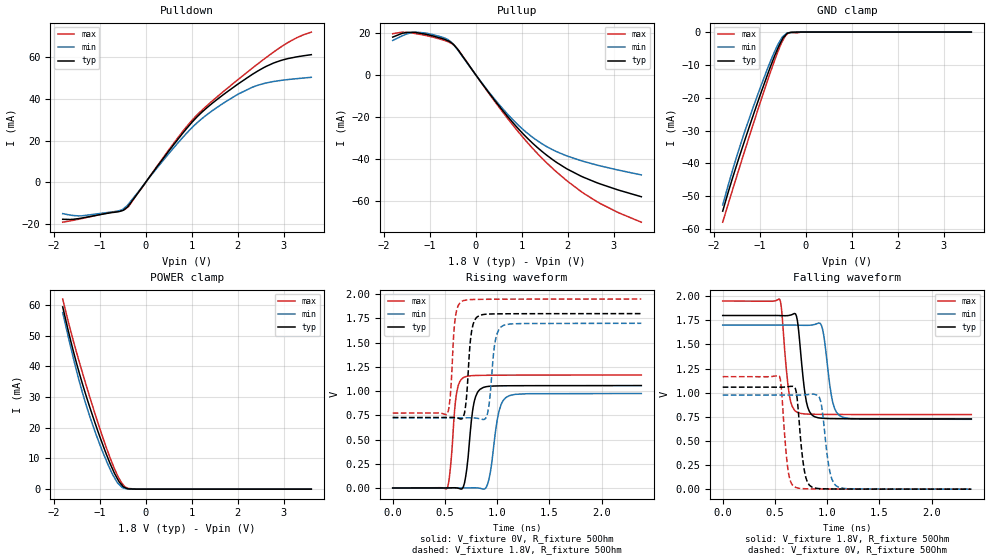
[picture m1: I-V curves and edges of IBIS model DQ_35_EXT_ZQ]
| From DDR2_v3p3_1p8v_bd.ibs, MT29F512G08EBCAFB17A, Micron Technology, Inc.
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| MODEL DQ_35_EXT_ZQ (35 Ohm Data I/O with no ODT, With ZQ Cal)
[Model]   DQ_35_EXT_ZQ
Model_type   I/O
Vinl = 650.000mV
Vinh = 1.150V
Vmeas = 900.000mV
Vref = 900.000mV
Cref = 0.0pF
Rref = 50.000Ohm
|   typ   min   max
|C_comp   1.200pF   1.100pF   1.300pF
C_comp_pullup   0.6000pF   0.5500pF   0.6500pF
C_comp_pulldown   0.6000pF   0.5500pF   0.6500pF
[Model Spec]
| Input threshold voltage corners
Vinl   0.6500V   0.6000V   0.7250V
Vinh   1.1500V   1.1000V   1.2250V
| Measurement voltage corners
Vmeas   0.9000V   0.8500V   0.9750V
| Timing spec test load voltage corners
Vref   0.9000V   0.8500V   0.9750V
| Dynamic Overshoot Parameters from ONFI4 Specification
D_overshoot_ampl_h   1.00   NA   NA
D_overshoot_ampl_l   1.00   NA   NA
D_overshoot_area_h   0.75n   NA   NA
D_overshoot_area_l   0.75n   NA   NA
[Receiver Thresholds]
Vth   =  0.900V
Vth_min  =  0.8820V
Vth_max  =  0.9180V
Vinh_ac  =  0.250V
Vinh_dc  =  0.125V
Vinl_ac  = -0.250V
Vinl_dc  = -0.125V
Tslew_ac =  5.000ns |Not specified, so set to high value
Threshold_sensitivity = 0.50
Reference_supply Pullup_ref
[Voltage Range]   1.8000V   1.7000V   1.9500V
[Pullup Reference]   1.8000V   1.7000V   1.9500V
| Junction Temperature (Ambient temp is 35C typ, 70C min, 0C max)
[Temperature Range]   50.0   85.0   0.0
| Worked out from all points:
|   slope of the pulldown table from 0 to 0.27 V, typ, clamps not added: 33.1 ohm
|   slope of the pullup table from 0 to 0.27 V, typ, clamps not added: 33.4 ohm
|   GND clamp passes 1 mA (typ) near -0.44 V on its own axis
|   POWER clamp passes 1 mA (typ) near -0.50 V on its own axis
|   falling waveform, V_fixture 1.8V, R_fixture 50Ohm: 20-80 % time 63.1ps typ, 71ps min, 58.7ps max; typ from 1.8 V to 0.728 V
|   rising waveform, V_fixture 0V, R_fixture 50Ohm: 20-80 % time 61.4ps typ, 75.9ps min, 51.1ps max; typ from 0 V to 1.06 V
|   rising waveform, V_fixture 1.8V, R_fixture 50Ohm: 20-80 % time 44.4ps typ, 51.4ps min, 39.1ps max; typ from 0.728 V to 1.8 V
|   falling waveform, V_fixture 0V, R_fixture 50Ohm: 20-80 % time 58ps typ, 66.3ps min, 52ps max; typ from 1.06 V to 0 V
[Pulldown]
|   Voltage   I(typ)   I(min)   I(max)
-1.8V     -17.7mA    -14.98mA   -19.1mA
-1.382V   -17.11mA   -16.04mA   -17.33mA
-608.3mV  -14.13mA   -13.83mA   -13.84mA
-442.8mV  -12.67mA   -11.96mA   -12.9mA
-362.9mV  -10.97mA   -10.16mA   -11.4mA
901.3mV   26.16mA    23.87mA    27.08mA
1.224V    33.76mA    30.65mA    34.67mA
1.548V    39.76mA    35.96mA    41mA
2.021V    47.48mA    42.52mA    49.64mA
2.623V    55.77mA    47.79mA    60.05mA
3.092V    59.47mA    49.4mA     67.19mA
3.6V      61.35mA    50.48mA    72.2mA
[GND Clamp]
|   Voltage   I(typ)   I(min)   I(max)
-1.8V     -54.56mA   -52.69mA   -57.93mA
-1.548V   -42.78mA   -40.31mA   -46.36mA
-1.327V   -33.25mA   -30.57mA   -36.44mA
-1.077V   -22.86mA   -20.51mA   -25.43mA
-817.4mV  -12.62mA   -10.81mA   -14.45mA
-608.3mV  -5.168mA   -3.972mA   -6.219mA
-520.8mV  -2.645mA   -1.885mA   -3.256mA
-480.6mV  -1.611mA   -1.209mA   -2.217mA
-442.8mV  -1.066mA   -762.6uA   -1.241mA
-364.8mV  -238.2uA   -221uA     -173.5uA
-163.8mV  -972.9nA   0A         -201.1uA
3.604V    0A         0A         0A
[Pullup]
|   Voltage   I(typ)   I(min)   I(max)
-1.8V     17.84mA    16.24mA    19.44mA
-1.297V   20mA       20.22mA    19.5mA
-713.7mV  17.06mA    17.72mA    16.51mA
-520.8mV  15.03mA    15.26mA    14.81mA
-362.9mV  11.26mA    10.99mA    11.39mA
574.9mV   -16.7mA    -15.87mA   -17.41mA
971mV     -26.78mA   -24.94mA   -28.36mA
1.333V    -34.51mA   -31.33mA   -37.32mA
1.765V    -41.86mA   -36.72mA   -46.45mA
2.338V    -48.79mA   -41.26mA   -56.33mA
3.067V    -54.69mA   -45.27mA   -65.33mA
3.6V      -58.12mA   -47.73mA   -70.22mA
[POWER Clamp]
|   Voltage   I(typ)   I(min)   I(max)
-1.8V     59.37mA    57.52mA    61.9mA
-1.585V   45.91mA    43.7mA     49.21mA
-1.437V   37.69mA    35mA       41.3mA
-1.276V   29.7mA     26.71mA    33.17mA
-1.077V   20.68mA    17.92mA    23.6mA
-871.2mV  12.13mA    9.982mA    14.37mA
-712mV    6.399mA    4.675mA    8.008mA
-572.4mV  2.368mA    1.496mA    3.424mA
-504.6mV  1.145mA    486.6uA    1.765mA
-442.8mV  468.7uA    231.8uA    685.7uA
-178.2mV  0A         0A         0A
3.604V    0A         0A         0A
[Ramp]
R_load = 50
|   typ   min   max
dV/dt_r 6.3425E-01/6.1156E-11   5.8519E-01/7.5395E-11   6.9956E-01/5.0656E-11
dV/dt_f 6.4316E-01/6.2537E-11   5.8549E-01/7.0593E-11   7.0614E-01/5.8457E-11
[Falling Waveform]
V_fixture = 1.8V
V_fixture_min = 1.7V
V_fixture_max = 1.95V
R_fixture = 50Ohm
C_fixture = 0F
|   Time   V(typ)   V(min)   V(max)
0s        1.8V       1.7V       1.95V
546ps     1.799V     1.7V       1.966V
636ps     1.801V     1.7V       988.7mV
714ps     1.751V     1.7V       796.6mV
800ps     911mV      1.698V     778.8mV
866ps     759.3mV    1.703V     776.4mV
956ps     734.8mV    1.658V     775.1mV
1.038ns   731.2mV    983.7mV    774.4mV
1.114ns   730mV      766.3mV    774.1mV
2.38ns    728.1mV    724.1mV    773.1mV
[Rising Waveform]
V_fixture = 0V
V_fixture_min = 0V
V_fixture_max = 0V
R_fixture = 50Ohm
C_fixture = 0F
|   Time   V(typ)   V(min)   V(max)
0s        77.71uV    148.8uV    25.96uV
520ps     407uV      108.2uV    -4.379mV
610ps     1.34mV     67.12uV    969.2mV
686ps     46.66mV    216.9uV    1.144V
778ps     879.3mV    2.279mV    1.161V
866ps     1.037V     -11.54mV   1.163V
932ps     1.05V      146.7mV    1.164V
1.018ns   1.054V     793.6mV    1.164V
1.082ns   1.055V     932.3mV    1.165V
2.38ns    1.057V     975.5mV    1.166V
[Rising Waveform]
V_fixture = 1.8V
V_fixture_min = 1.7V
V_fixture_max = 1.95V
R_fixture = 50Ohm
C_fixture = 0F
|   Time   V(typ)   V(min)   V(max)
0s        728mV      724mV      773.1mV
522ps     728.3mV    724mV      762.5mV
600ps     726.8mV    723.8mV    1.766V
670ps     720.2mV    723.9mV    1.931V
756ps     1.623V     724.3mV    1.945V
830ps     1.78V      715.4mV    1.947V
906ps     1.795V     763.3mV    1.948V
984ps     1.797V     1.529V     1.948V
1.064ns   1.798V     1.68V      1.949V
2.38ns    1.8V       1.7V       1.95V
[Falling Waveform]
|Gnd
V_fixture = 0V
V_fixture_min = 0V
V_fixture_max = 0V
R_fixture = 50Ohm
C_fixture = 0F
|   Time   V(typ)   V(min)   V(max)
0s        1.057V     975.6mV    1.166V
542ps     1.056V     975.7mV    1.172V
626ps     1.062V     975.7mV    195mV
696ps     1.04V      975.2mV    19.77mV
782ps     191.3mV    977mV      4.814mV
856ps     20.36mV    984.4mV    2.815mV
940ps     4.792mV    900.3mV    1.923mV
1.014ns   2.602mV    250.1mV    1.443mV
1.084ns   1.808mV    35.79mV    1.154mV
2.38ns    156.7uV    262.2uV    75.18uV
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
